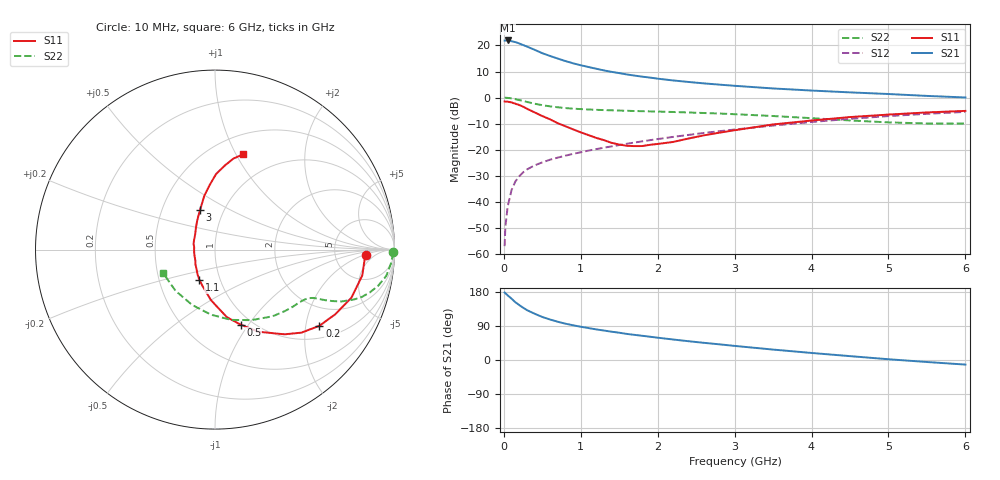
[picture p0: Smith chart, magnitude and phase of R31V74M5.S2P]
! SIEMENS Small Signal Semiconductors
! BFR181
! Si NPN RF Bipolar Junction Transistor in SOT23
! VCE = 1.75 V  IC = 4.5 mA
! Common Emitter S-Parameters:  May  1996
# GHz  S  MA  R  50
!  f  S11  S21  S12  S22
! GHz  MAG  ANG  MAG  ANG  MAG  ANG  MAG  ANG
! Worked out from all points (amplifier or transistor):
!   36 points, 10 MHz to 6 GHz, reference 50 ohm
!   highest |S21| = 21.9 dB at 50 MHz (marker M1)
!   |S21| within 3 dB of that: start of sweep to 353.1 MHz
!   unconditionally stable (mu >= 1): 1.122 GHz to 3.029 GHz
!   at 250 MHz: K = 0.40, MSG = 24.5 dB, |S12| = -28.8 dB
!   at 1.4 GHz: K = 1.05, MAG = 12.9 dB, |S12| = -18.8 dB
!   at 6 GHz: K = 0.86, MSG = 2.8 dB, |S12| = -5.5 dB
!   S11 on the Smith chart (normalised r, x): 10 MHz: 11, -2; 200 MHz: 1.36, -2.39; 500 MHz: 0.88, -0.92; 1.1 GHz: 0.80, -0.28; 3 GHz: 0.77, +0.36; 6 GHz: 0.70, +1.07
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0.01  0.8428 -2.2  12.44 178.2  0.0014 89.8  0.9923 -0.9
0.02  0.8355 -3.7  12.46 176.0  0.0033 87.5  0.9904 -1.8
0.05  0.8331 -10.0  12.48 170.6  0.0081 82.8  0.9839 -4.4
0.1  0.806 -19.4  12.06 161.9  0.0167 79.1  0.9658 -8.7
0.15  0.7612 -28.2  11.61 152.3  0.0245 74.4  0.931 -12.5
0.2  0.7202 -36.1  10.92 145.1  0.0307 71.5  0.8945 -15.5
0.25  0.6683 -43.8  10.2 138.1  0.0365 68.3  0.8606 -17.8
0.3  0.6108 -50.6  9.536 131.7  0.0416 67.1  0.8238 -19.7
0.4  0.5181 -62.1  8.262 122.1  0.0499 63.2  0.7617 -22.3
0.5  0.4414 -71.2  7.107 113.5  0.0569 62.0  0.7133 -23.7
0.6  0.3823 -80.0  6.288 106.9  0.0641 61.4  0.6778 -24.6
0.7  0.322 -87.4  5.612 101.0  0.0702 61.5  0.6503 -25.2
0.8  0.2811 -94.8  5.021 95.9  0.0765 60.9  0.6286 -25.7
1.1  0.1901 -117.2  3.859 84.3  0.0958 62.4  0.5897 -27.3
1.3  0.1522 -132.1  3.322 77.8  0.109 62.7  0.5743 -28.8
1.6  0.1185 -166.0  2.775 68.8  0.1297 63.0  0.5572 -31.5
2.2  0.1403 141.8  2.13 54.1  0.1756 61.9  0.5281 -38.8
3  0.2356 110.7  1.681 37.2  0.2433 57.4  0.4789 -51.8
3.5  0.3045 101.4  1.495 27.5  0.29 53.4  0.4417 -62.9
4.5  0.422 89.1  1.257 10.2  0.39 43.1  0.3631 -93.6
5.5  0.518 78.5  1.075 -5.3  0.4871 30.2  0.3178 -134.0
6  0.5545 73.4  1.003 -12.1  0.5307 23.1  0.3173 -155.8
